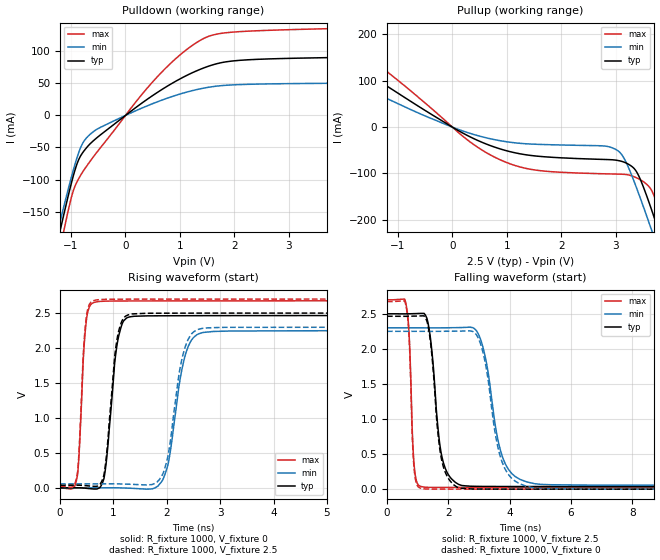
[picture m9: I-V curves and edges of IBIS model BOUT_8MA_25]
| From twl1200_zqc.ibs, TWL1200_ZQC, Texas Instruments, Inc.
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[Model]   BOUT_8MA_25
Model_type  Output
Vref =   2.5
Rref =   1M
Cref =   15p
Vmeas =   1.25
| variable   typ   min   max
C_comp   4.10pF   2.76pF   5.42pF
| C_pullup   4.40pF   2.76pF   5.42pF
| C_pulldown   3.79pF   3.03pF   4.93pF
[Temperature Range]   40   100   -40
| Ambient temperature   25   85   -40
[Voltage range]   2.5   2.3   2.7
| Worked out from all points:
|   slope of the pulldown table from 0 to 0.375 V, typ, clamps not added: 15.8 ohm
|   slope of the pullup table from 0 to 0.375 V, typ, clamps not added: 15.8 ohm
|   rising waveform, R_fixture 1000, V_fixture 0: 20-80 % time 171ps typ, 262ps min, 101ps max; typ from 0 V to 2.46 V
|   falling waveform, R_fixture 1000, V_fixture 2.5: 20-80 % time 306ps typ, 513ps min, 127ps max; typ from 2.5 V to 0.037 V
|   rising waveform, R_fixture 1000, V_fixture 2.5: 20-80 % time 167ps typ, 252ps min, 99.2ps max; typ from 0.037 V to 2.5 V
|   falling waveform, R_fixture 1000, V_fixture 0: 20-80 % time 300ps typ, 502ps min, 124ps max; typ from 2.46 V to 0 V
[Pulldown]
| BOUT_8MA_25
|   Voltage   I(typ)   I(min)   I(max)
-2.5V     -690.3mA   -641.5mA   -763mA
-1.245V   -196.5mA   -181mA     -226.5mA
-1.19V    -175.8mA   -161.9mA   -203.6mA
-1.14V    -157.3mA   -144.7mA   -183.2mA
-970mV    -98.03mA   -88.92mA   -120.7mA
-885mV    -74.36mA   -64.43mA   -102.6mA
-770mV    -56.23mA   -41.12mA   -86.03mA
-620mV    -41.83mA   -27.27mA   -68.05mA
575mV     35.31mA    20.91mA    59.4mA
1.43V     73.88mA    42.51mA    119.8mA
2.255V    86.85mA    48.56mA    131.5mA
5V        91.85mA    50.86mA    137.9mA
[Pullup]
| BOUT_8MA_25
|   Voltage   I(typ)   I(min)   I(max)
-2.5V     182.5mA    132.1mA    229mA
-1.685V   124.1mA    87.9mA     162.9mA
85mV      -5.859mA   -3.785mA   -8.983mA
775mV     -43.04mA   -26.99mA   -64.67mA
1.54V     -62.39mA   -36.98mA   -92.85mA
2.945V    -70.5mA    -44.99mA   -101.1mA
3.13V     -74.54mA   -62.43mA   -101.7mA
3.345V    -89.98mA   -119mA     -107.3mA
3.65V     -174.9mA   -218.7mA   -134.3mA
3.76V     -213.2mA   -256.3mA   -165.3mA
3.895V    -261.6mA   -303.2mA   -213.5mA
5V        -678.1mA   -700.7mA   -652.5mA
[Ramp]
| BOUT_8MA_25
| variable   typ   min   max
dV/dt_r   1.49/1.93E-10   1.36/2.72E-10   1.61/1.10E-10
dV/dt_f   1.48/3.21E-10   1.35/5.20E-10   1.61/1.30E-10
R_load = 1000
[Rising Waveform]
| BOUT_8MA_25
R_fixture =   1000
C_fixture =   0
L_fixture =   0
V_fixture =   0
V_fixture_min = 0
V_fixture_max = 0
|   Time   V(typ)   V(min)   V(max)
0s        8.384nV    35.52nV    717pV
325ps     1.37mV     -24.3uV    184.4mV
520ps     -8.176mV   -48.55uV   2.523V
820ps     130.5mV    1.236mV    2.669V
945ps     1.052V     1.819mV    2.671V
1.24ns    2.425V     -2.688mV   2.673V
1.935ns   2.461V     134.9mV    2.674V
2.465ns   2.462V     2.117V     2.674V
3.19ns    2.463V     2.243V     2.675V
238.2ns   2.465V     2.25V      2.675V
[Falling Waveform]
| BOUT_8MA_25
R_fixture =   1000
C_fixture =   0
L_fixture =   0
V_fixture =   2.5
V_fixture_min = 2.3
V_fixture_max = 2.7
|   Time   V(typ)   V(min)   V(max)
0s        2.5V       2.3V       2.7V
600ps     2.499V     2.3V       2.676V
720ps     2.5V       2.3V       2.204V
910ps     2.502V     2.3V       235.1mV
1.335ns   2.375V     2.299V     25.94mV
1.84ns    374.3mV    2.3V       24.61mV
2.84ns    40.78mV    2.291V     23.95mV
3.86ns    37.96mV    357.8mV    23.71mV
5.34ns    37.41mV    63.11mV    23.59mV
238.2ns   37.17mV    56.86mV    23.53mV
[Rising Waveform]
| BOUT_8MA_25
R_fixture =   1000
C_fixture =   0
L_fixture =   0
V_fixture =   2.5
V_fixture_min = 2.3
V_fixture_max = 2.7
|   Time   V(typ)   V(min)   V(max)
0s        37.17mV    56.86mV    23.53mV
325ps     38.39mV    56.84mV    217.6mV
520ps     29.09mV    56.82mV    2.564V
895ps     687.6mV    58.37mV    2.697V
1.045ns   2.016V     57.8mV     2.698V
1.21ns    2.445V     54.49mV    2.698V
1.89ns    2.498V     151.5mV    2.699V
2.38ns    2.499V     2.092V     2.699V
3.075ns   2.499V     2.296V     2.7V
238.2ns   2.5V       2.3V       2.7V
[Falling Waveform]
| BOUT_8MA_25
R_fixture =   1000
C_fixture =   0
L_fixture =   0
V_fixture =   0
V_fixture_min = 0
V_fixture_max = 0
|   Time   V(typ)   V(min)   V(max)
0s        2.465V     2.25V      2.675V
620ps     2.464V     2.25V      2.61V
720ps     2.465V     2.25V      2.166V
905ps     2.467V     2.25V      205.4mV
1.315ns   2.373V     2.249V     2.233mV
1.83ns    331.4mV    2.251V     990.1uV
2.76ns    3.545mV    2.252V     417.4uV
3.84ns    707uV      295.9mV    175.8uV
5.255ns   237.9uV    5.986mV    63.05uV
238.2ns   19.88nV    53.75nV    5.96nV
